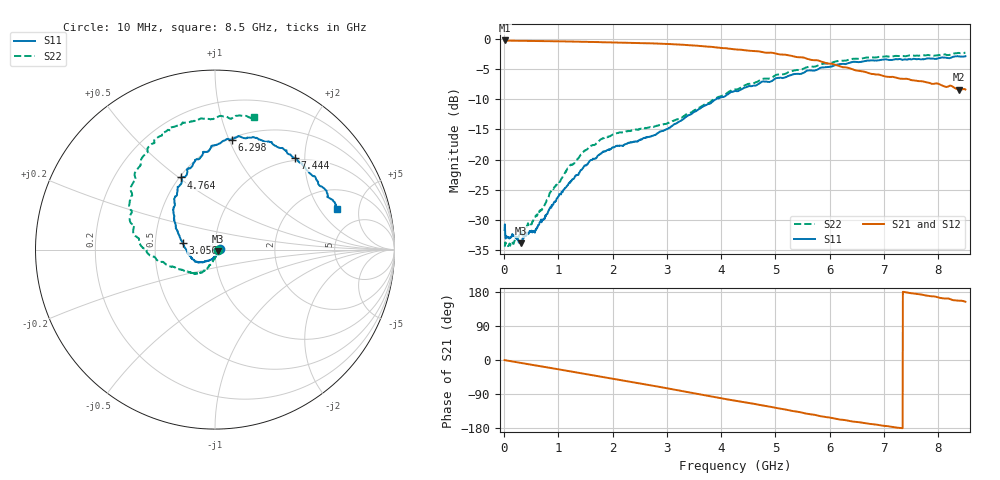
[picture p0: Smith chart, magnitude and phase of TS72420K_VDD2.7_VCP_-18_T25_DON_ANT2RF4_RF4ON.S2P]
!Agilent Technologies,E5071C,MY46417908,A.11.23
!Date: Thu Oct 03 16:41:53 2019
!Data & Calibration Information:
!Freq	S11:SOLT2(ON)	S21:SOLT2(ON)	S12:SOLT2(ON)	S22:SOLT2(ON)
!PortZ  Port1:50+j0  Port2:50+j0
!Above PortZ is port z conversion or system Z0 setting when saving the data.
!When reading, reference impedance value at option line is always used.
# Hz S dB R 50
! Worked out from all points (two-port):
!   1601 points, 10 MHz to 8.5 GHz, reference 50 ohm
!   highest |S21| = -0.26 dB at 10 MHz (marker M1); lowest = -8.4 dB at 8.389 GHz (marker M2)
!   |S21| within 3 dB of the highest: start of sweep to 5.575 GHz
!   lowest |S11| = -33.9 dB at 317.8 MHz (marker M3), VSWR 1.04, Z = 51.7 - j1.09 ohm
!   |S11| at or under -10 dB: start of sweep to 3.903 GHz
!   |S22| runs from -34.4 to -2.3 dB; largest |S21 - S12| = 0.0067
!   S11 on the Smith chart (normalised r, x): 10 MHz: 1.05, +0.01; 3.056 GHz: 0.69, +0.06; 4.764 GHz: 0.51, +0.51; 6.298 GHz: 0.51, +1.02; 7.444 GHz: 0.95, +1.80; 8.5 GHz: 3.20, +2.96
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1e7  -31.69 5.8  -0.26 -0.3  -0.25 -0.3  -34.24 -8.3
6.836875e7  -32.94 -9.6  -0.29 -1.8  -0.27 -1.8  -34.29 -16.7
1.532688e8  -32.36 -13.5  -0.31 -3.9  -0.29 -3.9  -33.87 -25.2
3.177625e8  -33.89 -31.4  -0.33 -7.9  -0.31 -8.0  -31.92 -40.8
5.83075e8  -31.59 -71.0  -0.36 -14.4  -0.35 -14.4  -29.32 -74.6
1.187988e9  -23.98 -115.1  -0.43 -29.1  -0.43 -29.1  -21.32 -106.8
1.426769e9  -21.70 -127.8  -0.48 -35.0  -0.48 -35.0  -19.15 -112.1
1.851269e9  -18.68 -142.2  -0.56 -45.4  -0.56 -45.4  -16.40 -122.2
2.843538e9  -15.54 177.1  -0.79 -70.4  -0.78 -70.5  -14.36 -138.6
3.055788e9  -14.67 167.6  -0.86 -76.0  -0.85 -76.1  -13.80 -143.9
3.597025e9  -11.61 147.1  -1.16 -90.4  -1.15 -90.4  -11.41 -159.8
4.255e9  -8.63 127.0  -1.75 -107.2  -1.73 -107.2  -8.40 -178.9
4.7644e9  -7.06 115.1  -2.20 -120.0  -2.17 -120.0  -6.62 167.8
5.268494e9  -6.06 103.9  -2.76 -133.2  -2.71 -133.0  -5.41 153.3
5.671769e9  -5.23 96.0  -3.50 -143.7  -3.46 -143.4  -4.60 139.6
6.297906e9  -4.16 81.5  -4.72 -158.9  -4.73 -158.8  -3.60 124.5
6.7171e9  -3.58 70.9  -5.67 -168.3  -5.67 -168.2  -3.08 117.3
7.088538e9  -3.49 60.8  -6.29 -175.1  -6.27 -174.5  -2.94 111.0
7.444056e9  -3.38 48.9  -6.66 177.5  -6.66 178.0  -2.79 104.7
7.788962e9  -3.25 36.5  -7.21 170.0  -7.25 170.1  -2.70 96.6
8.388569e9  -2.91 19.9  -8.41 156.5  -8.43 156.3  -2.34 76.4
8.5e9  -2.88 18.2  -8.39 153.6  -8.37 153.1  -2.26 73.6
